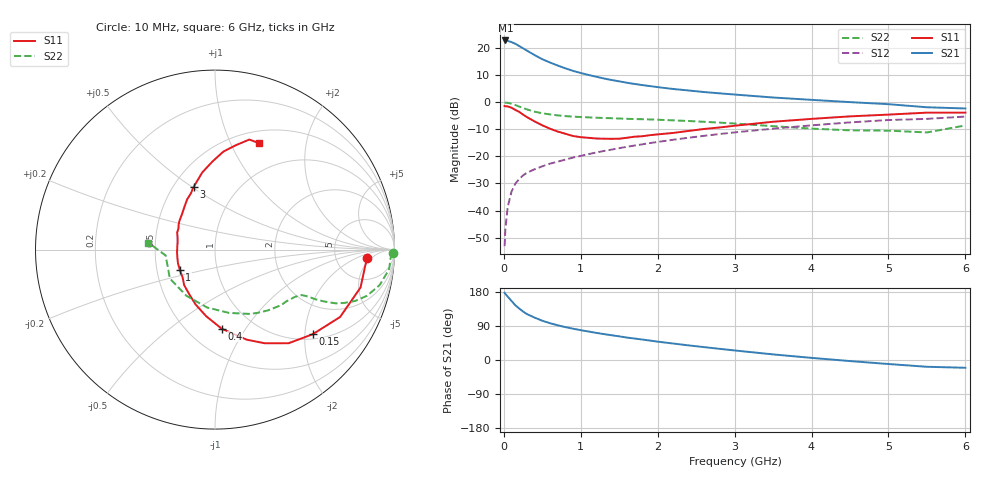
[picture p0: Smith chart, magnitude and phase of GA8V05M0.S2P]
! Infineon Technologies  Discrete & RF Semiconductors
! BF775
! Si NPN RF Bipolar Junction Transistor in SOT23
! VCE = 8 V  IC = 5 mA
! Common Emitter S-Parameters:  May  1996
# GHz  S  MA  R  50
!  f  S11  S21  S12  S22
! GHz  MAG  ANG  MAG  ANG  MAG  ANG  MAG  ANG
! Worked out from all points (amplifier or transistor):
!   36 points, 10 MHz to 6 GHz, reference 50 ohm
!   highest |S21| = 22.8 dB at 20 MHz (marker M1)
!   |S21| within 3 dB of that: start of sweep to 255.2 MHz
!   unconditionally stable (mu >= 1): 846.2 MHz to 3.022 GHz
!   at 250 MHz: K = 0.47, MSG = 23.5 dB, |S12| = -27.0 dB
!   at 1.4 GHz: K = 1.10, MAG = 10.9 dB, |S12| = -17.5 dB
!   at 6 GHz: K = 0.90, MSG = 1.5 dB, |S12| = -5.3 dB
!   lowest NFmin = 1.50 dB at 450 MHz
!   S11 on the Smith chart (normalised r, x): 10 MHz: 11, -4; 150 MHz: 1.12, -2.19; 400 MHz: 0.72, -0.79; 1 GHz: 0.66, -0.16; 3 GHz: 0.63, +0.51; 6 GHz: 0.64, +1.29
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0.01  0.8505 -3.1  13.8 177.2  0.0022 89.5  0.9932 -1.2
0.02  0.8421 -6.0  13.81 174.4  0.0046 87.6  0.9798 -2.6
0.05  0.8379 -14.6  13.58 167.3  0.0116 82.3  0.9762 -6.4
0.1  0.7918 -28.3  12.87 155.8  0.0224 75.8  0.9391 -12.1
0.15  0.7203 -40.9  12 144.3  0.0314 69.4  0.8853 -16.9
0.2  0.6637 -51.8  10.89 135.8  0.0383 65.6  0.832 -20.1
0.25  0.5911 -62.0  9.879 127.9  0.0445 61.9  0.7821 -22.3
0.3  0.5321 -70.6  8.976 121.2  0.0499 60.4  0.7367 -24.0
0.4  0.442 -85.2  7.415 111.9  0.0579 58.5  0.6696 -25.5
0.5  0.3745 -97.5  6.218 103.6  0.0656 57.6  0.6254 -26.3
0.6  0.3249 -109.3  5.406 97.1  0.0733 57.6  0.5951 -26.6
0.8  0.2618 -131.1  4.219 86.8  0.0873 58.4  0.5543 -27.4
1  0.2263 -149.9  3.46 78.7  0.1021 59.2  0.5333 -28.7
1.1  0.2201 -159.6  3.191 75.2  0.11 59.5  0.5251 -29.7
1.3  0.212 -175.8  2.746 68.4  0.126 59.4  0.5117 -31.5
1.6  0.2209 161.0  2.291 59.2  0.1504 59.1  0.494 -35.2
2.2  0.2709 132.5  1.756 43.5  0.2027 56.5  0.4626 -44.7
3  0.3679 109.0  1.386 25.2  0.2774 50.1  0.4045 -62.3
3.5  0.4363 99.3  1.222 14.8  0.3248 44.8  0.3613 -77.5
4.5  0.5481 85.1  1.005 -2.8  0.4244 32.9  0.3025 -121.7
5.5  0.6422 72.7  0.807 -17.9  0.4927 17.5  0.2768 -173.2
6  0.642 67.5  0.767 -20.5  0.5436 13.2  0.3726 174.1
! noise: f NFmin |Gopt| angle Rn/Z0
0.45  1.5  0.28  29  0.34
0.9  1.8  0.25  59  0.34
